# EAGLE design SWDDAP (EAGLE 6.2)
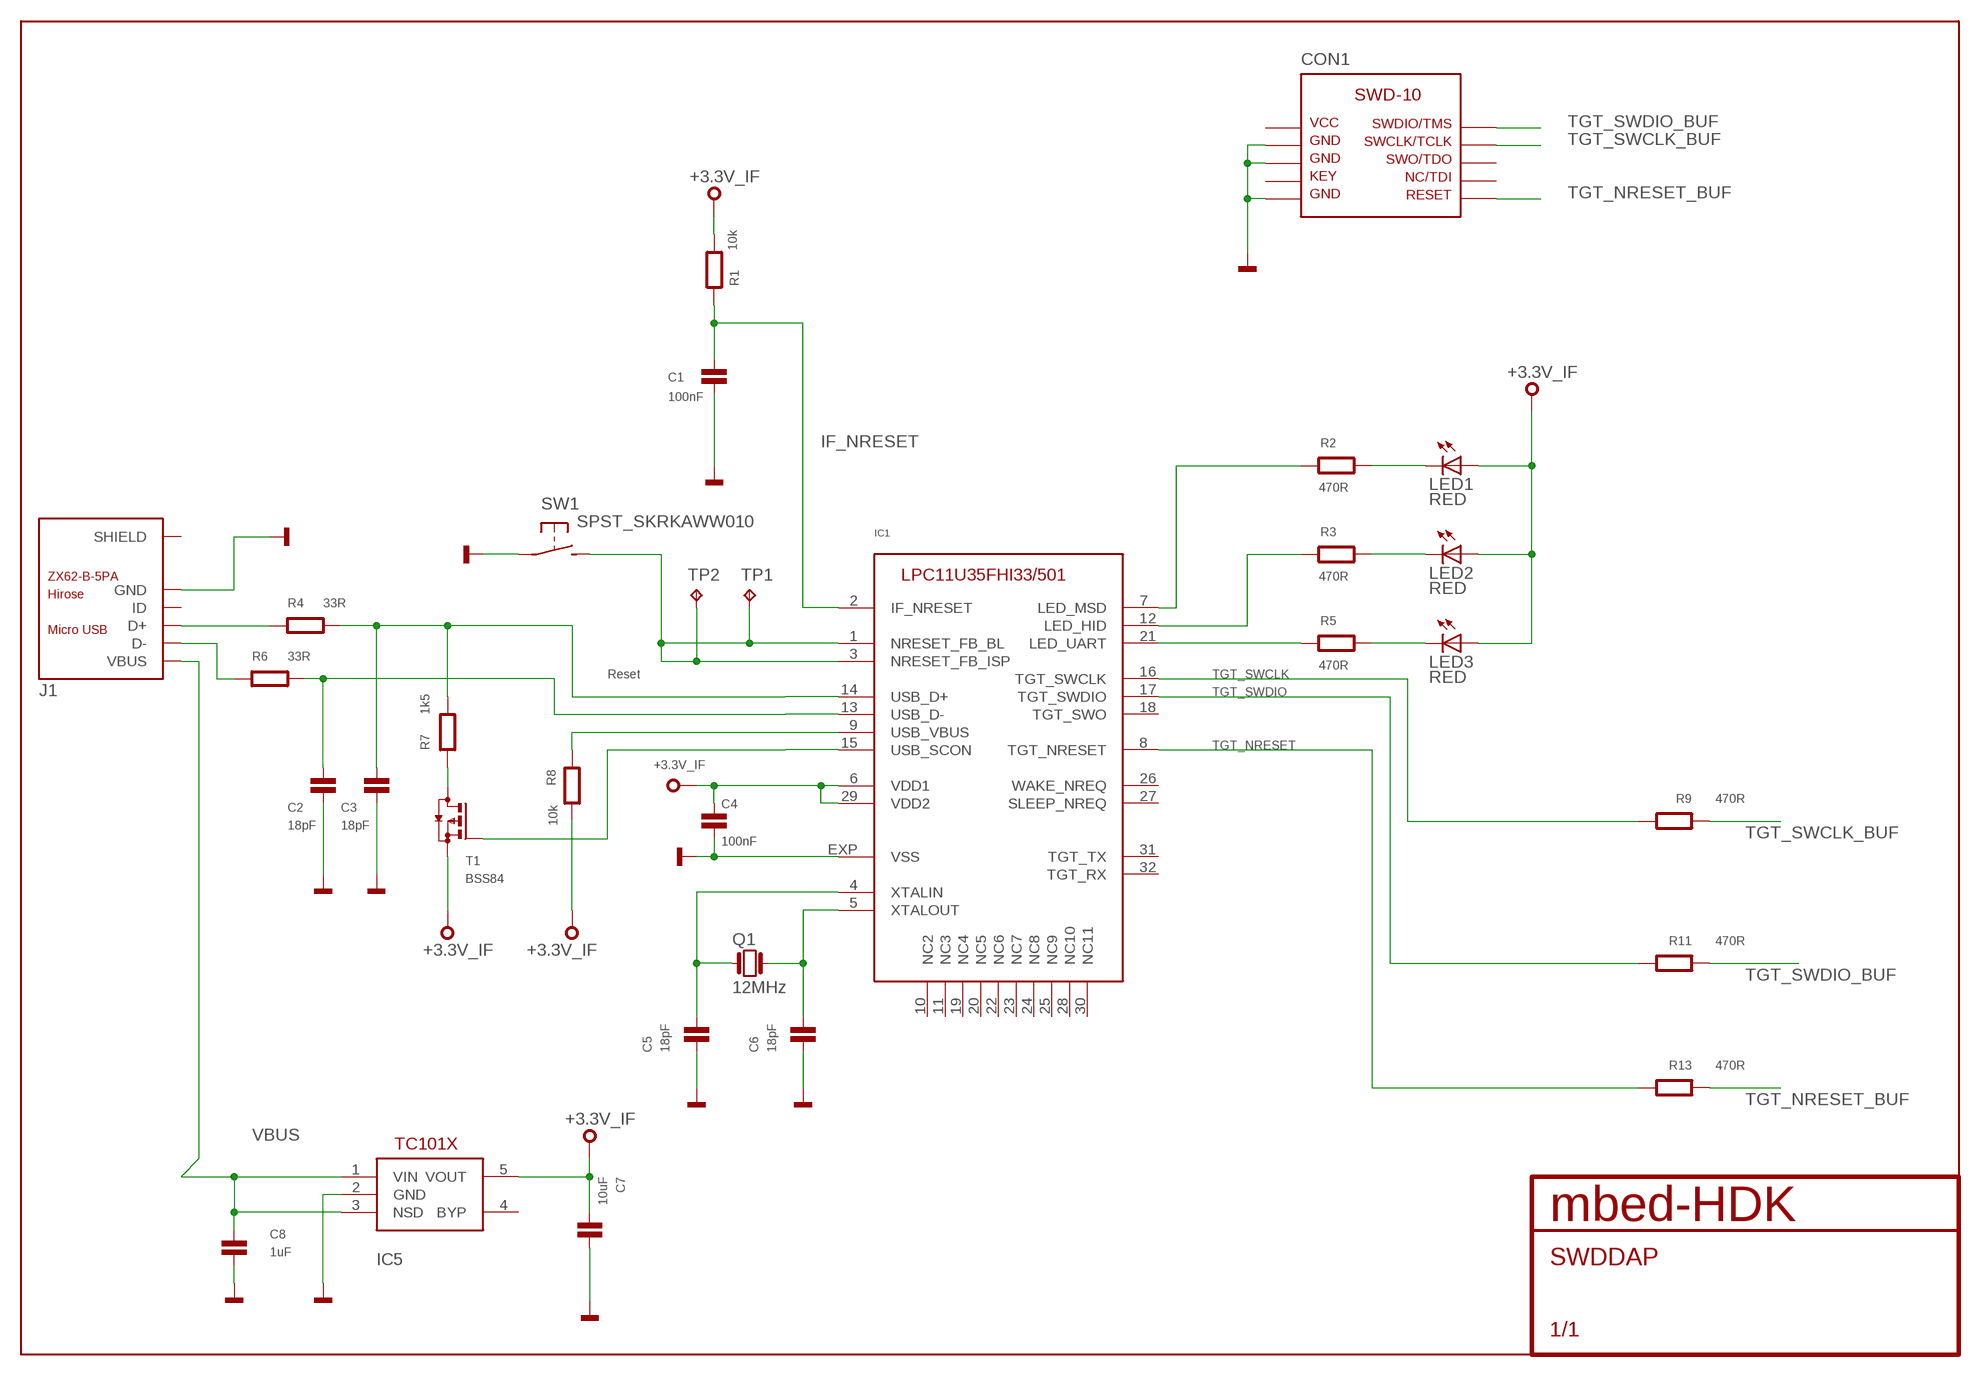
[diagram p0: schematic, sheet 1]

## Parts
C1  100nF  C0402  [0402]
C2  18pF  C0402  [0402]
C3  18pF  C0402  [0402]
C4  100nF  C0402  [0402]
C5  18pF  C0402  [0402]
C6  18pF  C0402  [0402]
C7  10uF  C0603  [0603]
C8  1uF  C0402  [0402]
CON1  SWD-10_SMD  [SWD-10-SMD]
IC1  IF-LPC11U35  [HVQFN33]
IC5  TC1014  [SOT23-5]
J1  ZX62-B-5PA  [ZX62-B-5PA(11)]
LED1  RED  LED0603  [CHIPLED_0603]
LED2  RED  LED0603  [CHIPLED_0603]
LED3  RED  LED0603  [CHIPLED_0603]
Q1  12MHz  Q_3.2X2.5  [3.2X.2.5]
R1  10k  R0402  [0402]
R2  470R  R0402  [0402]
R3  470R  R0402  [0402]
R4  33R  R0402  [0402]
R5  470R  R0402  [0402]
R6  33R  R0402  [0402]
R7  1k5  R0402  [0402]
R8  10k  R0402  [0402]
R9  470R  R0402  [0402]
R11  470R  R0402  [0402]
R13  470R  R0402  [0402]
SW1  SPST_SKRKAWW010  [SKRKAEE010]
T1  BSS84  [SOT23]
TP1  TPTP08SQ  [TP08SQ]
TP2  TPTP08SQ  [TP08SQ]

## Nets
+3,3V: C4.1 C7.2 IC1.6(VDD1) IC1.29(VDD2) IC5.5(VOUT) LED1.A LED2.A LED3.A R1.2 R8.2 T1.2(S) ; supply symbol labelled +3.3V_IF
GND: C1.2 C2.2 C3.2 C4.2 C5.2 C6.2 C7.1 C8.1 CON1.P$3 CON1.P$5 CON1.P$9 IC1.EXP(VSS) IC5.2(GND) J1.5(GND) SW1.P$1(P)
HID: IC1.12(LED_HID) R3.2
IF_NRESET: C1.1 IC1.2(IF_NRESET) R1.1
ISP: IC1.1(NRESET_FB_BL) IC1.3(NRESET_FB_ISP) SW1.P$2(S) TP1.TP TP2.TP
MSD: IC1.7(LED_MSD) R2.2
N$1: C3.1 IC1.14(USB_D+) R4.2 R7.2
N$2: C2.1 IC1.13(USB_D-) R6.2
N$3: J1.2(D-) R6.1
N$4: J1.3(D+) R4.1
N$5: LED1.C R2.1
N$6: R7.1 T1.3(D)
N$7: IC1.9(USB_VBUS) R8.1
N$8: LED2.C R3.1
N$9: LED3.C R5.1
N$12: C6.1 IC1.5(XTALOUT) Q1.P$3
N$14: C5.1 IC1.4(XTALIN) Q1.P$1
N$19: IC1.15(USB_SCON) T1.1(G)
TGT_NRESET: IC1.8(TGT_NRESET) R13.2
TGT_NRESET_BUF: CON1.P$10 R13.1
TGT_SWCLK: IC1.16(TGT_SWCLK) R9.2
TGT_SWCLK_BUF: CON1.P$4 R9.1
TGT_SWDIO: IC1.17(TGT_SWDIO) R11.2
TGT_SWDIO_BUF: CON1.P$2 R11.1
UART: IC1.21(LED_UART) R5.2
VBUS: C8.2 IC5.1(VIN) IC5.3(NSD) J1.1(VBUS)
Unconnected: CON1.P$1 CON1.P$6 CON1.P$7 CON1.P$8 IC1.10(NC2) IC1.11(NC3) IC1.18(TGT_SWO) IC1.19(NC4) IC1.20(NC5) IC1.22(NC6) IC1.23(NC7) IC1.24(NC8) IC1.25(NC9) IC1.26(WAKE_NREQ) IC1.27(SLEEP_NREQ) IC1.28(NC10) IC1.30(NC11) IC1.31(TGT_TX) IC1.32(TGT_RX) IC5.4(BYP) J1.4(ID) J1.SH1(SHIELD) J1.SH2(SHIELD) J1.SH3(SHIELD) J1.SH4(SHIELD) J1.SH5(SHIELD) J1.SH6(SHIELD)

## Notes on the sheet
- Reset

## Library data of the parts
C1-C8 = mbed-HDK:C: Capacitor
CON1 = mbed-HDK:SWD-10
IC1 = mbed-HDK:IF-LPC11U35
IC5 = Karasouli:TC1014
J1 = hirose:ZX62-B-5PA
LED1-LED3 = mbed-HDK:LED: SMD LED
Q1 = mbed-HDK:Q
R1-R9 R11 R13 = mbed-HDK:R
SW1 = mbed-switches:SPST
T1 = mbed-HDK:BSS84: P-CHANNEL MOS FET
TP1 TP2 = testpad:TP: Test pad

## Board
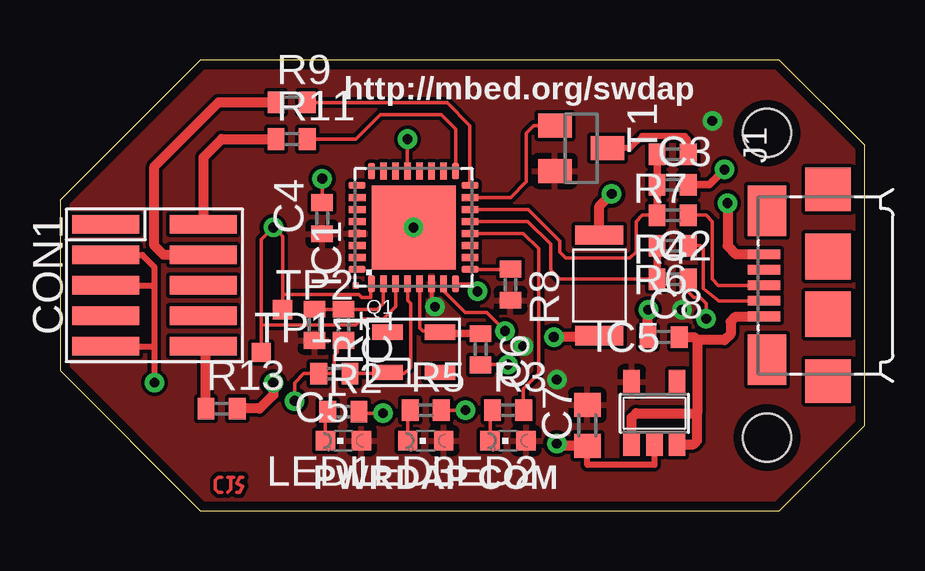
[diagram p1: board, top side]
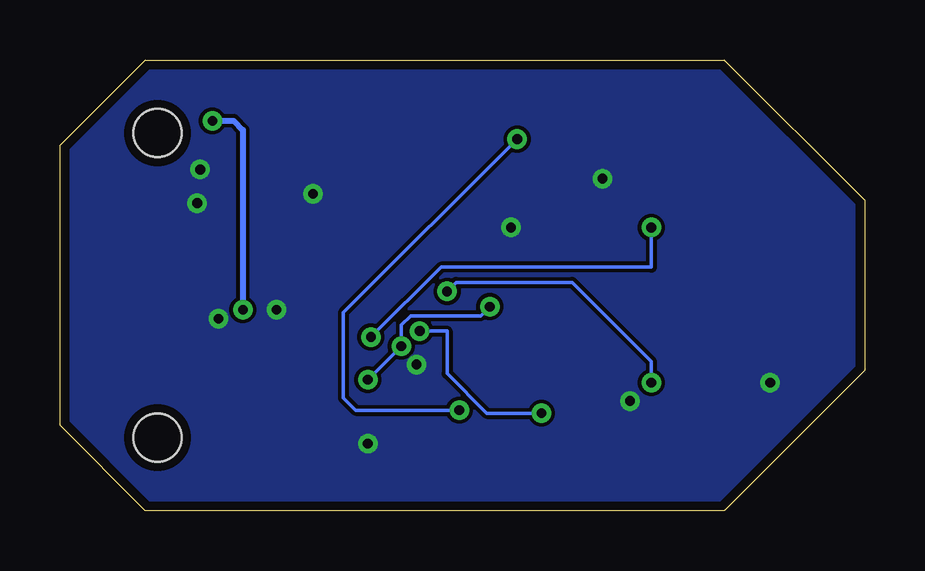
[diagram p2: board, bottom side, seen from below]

Size 33.53 x 18.8 mm. Coordinates in mm from the lower left corner, seen from the top.
Outline: 33.53,3.56 33.53,15.24 29.97,18.8 5.84,18.8 0,12.95 0,5.84 5.84,0 29.97,0 33.53,3.56
Copper layers (1*16): Top 0.035mm / dielectric 1.5mm / Bottom 0.035mm
Design rules: minimum track width 6mil, minimum drill 15mil, track to track 6mil, track to pad 6mil, pad to pad 6mil, via to via 6mil, smd to smd 6mil, copper to edge 15mil, drill to drill 8mil, minimum pad ring 10mil, minimum via ring 8mil, stop-mask expansion 4mil, vias tented up to drill 0mil, thermal gap 10mil
Holes 2 mm at 29.46,3.05 29.46,15.75

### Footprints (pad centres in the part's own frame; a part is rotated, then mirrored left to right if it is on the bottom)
0402 = smd 0.7 x 0.9: 1 -0.65,0; 2 0.65,0
0603 = smd 1 x 1.1: 1 -0.85,0; 2 0.85,0
SWD-10-SMD = smd 0.762 x 2.794: P$1 0.381,-2.032; P$2 0.381,2.032; P$3 1.651,-2.032; P$4 1.651,2.032; P$5 2.921,-2.032; P$6 2.921,2.032; P$7 4.191,-2.032; P$8 4.191,2.032; P$9 5.461,-2.032; P$10 5.461,2.032
HVQFN33 = smd 0.7 x 0.28: 1 -2.35,1.75; 2 -2.35,1.25; 3 -2.35,0.75; 4 -2.35,0.25; 5 -2.35,-0.25; 6 -2.35,-0.75; 7 -2.35,-1.25; 8 -2.35,-1.75; 17 2.35,-1.75; 18 2.35,-1.25; 19 2.35,-0.75; 20 2.35,-0.25; 21 2.35,0.25; 22 2.35,0.75; 23 2.35,1.25; 24 2.35,1.75 | smd 0.28 x 0.7: 9 -1.75,-2.35; 10 -1.25,-2.35; 11 -0.75,-2.35; 12 -0.25,-2.35; 13 0.25,-2.35; 14 0.75,-2.35; 15 1.25,-2.35; 16 1.75,-2.35; 25 1.75,2.35; 26 1.25,2.35; 27 0.75,2.35; 28 0.25,2.35; 29 -0.25,2.35; 30 -0.75,2.35; 31 -1.25,2.35; 32 -1.75,2.35 | smd 3.5 x 3.5: EXP 0,0 | smd 0.25 x 0.25: M1 -2.415,2.415
SOT23-5 = smd 0.69 x 0.99: 1 -0.95,-1.29; 2 0,-1.29; 3 0.95,-1.29; 4 0.95,1.3; 5 -0.95,1.3
ZX62-B-5PA(11) = smd 0.4 x 1.35: 1 -1.3,2.675; 2 -0.65,2.675; 3 0,2.675; 4 0.65,2.675; 5 1.3,2.675 | smd 2.1 x 1.6: SH1 -3.1,2.55; SH2 3.1,2.55 | smd 1.8 x 1.9: SH3 -4,0; SH6 4,0 | smd 1.9 x 1.9: SH4 -1.2,0; SH5 1.2,0
CHIPLED_0603 = smd 0.8 x 0.8: A 0,-0.75; C 0,0.75
3.2X.2.5 = smd 1.27 x 0.635: P$1 -1.092,-0.838; P$2 1.092,-0.838; P$3 1.092,0.838; P$4 -1.092,0.838
SKRKAEE010 = smd 0.8 x 2: P$1 -2.1,0; P$2 2.1,0
SOT23 = smd 1 x 1.4: 1 -0.95,-1.1; 2 0.95,-1.1; 3 0,1.1
TP08SQ = smd 0.8 x 0.8: TP 0,0

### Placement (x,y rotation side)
C1  11.81,7.75 270 top
C2  25.53,9.65 0 top
C3  25.53,13.59 0 top
C4  10.92,12.19 90 top
C5  11.43,5.71 180 top
C6  17.53,6.73 270 top
C7  21.97,3.56 90 top
C8  25.15,7.24 0 top
CON1  3.94,12.32 270 top
IC1  14.73,11.81 90 top
IC5  24.77,4.06 0 top
J1  32,9.4 90 top
LED1  11.81,2.92 90 top
LED2  18.67,2.92 90 top
LED3  15.24,2.92 90 top
Q1  14.73,6.6 0 top
R1  10.6,7.75 270 top
R2  11.81,4.13 0 top
R3  18.67,4.19 0 top
R4  25.53,12.32 180 top
R5  15.24,4.19 0 top
R6  25.53,11.05 180 top
R7  25.53,14.86 180 top
R8  18.77,9.42 270 top
R9  9.65,17.02 0 top
R11  9.65,15.49 0 top
R13  6.73,4.25 0 top
SW1  22.48,9.4 270 top
T1  21.72,15.11 270 top
TP1  8.38,6.6 0 top
TP2  9.27,8.38 0 top

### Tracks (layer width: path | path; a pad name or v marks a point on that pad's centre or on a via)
+3,3V  (via drill 0.41)
  Top 0.152: IC1.6 15.48,8.65 v15.62,8.51
  Bottom 0.152: v15.62,8.51 16,8.13 18.92,8.13 19.3,7.75 v19.3,6.86 v20.7,5.46
  Bottom 0.254: v27.18,16.26 26.29,16.26 25.91,15.88 v25.91,8.38
  pour Top: -5.08,19.18 -5.08,-0.25 34.54,-0.25 34.54,19.18
GND  (via drill 0.41)
  Top 0.152: C1.2 11.56,6.84 11.56,6.6 11.43,6.48 11.43,5.84 11.3,5.71 C5.2 10.16,5.71 9.78,5.33 v9.78,4.57 | C4.2 v10.92,13.84 10.68,14.08 | C6.2 17.54,6.1 v18.67,6.1 | C2.2 26.18,9.13 26.42,8.89 26.67,8.89 26.92,8.64 v26.92,8
  Top 0.254: IC5.2 24.77,1.9 21.97,1.9 C7.1 | CON1.P$3 3.43,10.67 3.94,10.16 3.94,9.4 | 3.94,9.4 3.94,6.86 | 3.94,6.86 v3.94,5.33 | CON1.P$9 3.94,6.86 | CON1.P$5 3.94,9.4
  Top 0.305: v27.69,14.22 27.05,13.59 C3.2
  Top 0.406: C7.1 20.7,2.71 v20.7,2.79 | C7.1 22.1,2.71 | 22.01,2.67 C7.1 | C8.1 24.5,8.37 v24.51,8.38 | 27.81,14.1 v27.69,14.22 | v27.81,12.83 27.81,11.05 28.16,10.7 J1.5 | SW1.P$1 22.48,12.7 v22.99,13.21
  other vias: 14.73,11.81
  pour Bottom: -5.08,-0.25 34.54,-0.25 34.54,19.18 -5.08,19.18
HID
  Top 0.152: IC1.12 19.3,11.56 19.94,10.92 19.94,5.71 19.3,5.08 19.3,4.21 R3.2
IF_NRESET
  Top 0.152: R1.1 C1.1 13.22,8.4 13.46,8.64 13.46,9.44 IC1.2
ISP  (via drill 0.41)
  Top 0.152: IC1.1 12.95,9.46 12.95,8.89 12.57,8.89 12.45,9.02 9.27,9.02 | IC1.3 13.98,8.52 13.46,8 12.57,8 12.32,7.75 8.38,7.75 | 8.38,7.75 8.38,11.3 v8.89,11.81 9.27,11.43 9.27,9.02 | TP1.TP 8.38,7.75 | TP2.TP 9.27,9.02
  Top 0.406: SW1.P$2 22.42,7.24 v20.57,7.24
  Bottom 0.152: v8.89,11.81 8.89,10.16 17.65,10.16 v20.57,7.24
MSD  (via drill 0.41)
  Top 0.152: IC1.7 15.98,9.16 16.89,8.25 17.78,8.25 v18.54,7.49 | v13.46,4.06 12.53,4.06 R2.2
  Bottom 0.152: v18.54,7.49 17.4,7.49 17.4,5.71 15.75,4.06 v13.46,4.06
N$1
  Top 0.152: IC1.14 19.51,12.56 20.83,11.24 20.83,10.79 21.08,10.54 23.75,10.54 24,10.79 24,12.06 24.26,12.32 R4.2
  Top 0.305: R4.2 C3.1 R7.2
N$2
  Top 0.152: IC1.13 19.5,12.06 20.45,11.11 20.45,10.03 20.83,9.65 C2.1
  Top 0.305: R6.2 C2.1
N$3
  Top 0.152: R6.1 26.67,11.05 26.8,10.92 26.8,9.91 26.8,9.78 26.8,9.27 27.43,8.76 27.45,8.75 J1.2
N$4
  Top 0.152: R4.1 26.92,12.32 27.18,12.06 27.18,9.65 27.43,9.4 J1.3
N$5
  Top 0.152: LED1.C 11.06,3.9 R2.1
N$6
  Top 0.254: R7.1 26.18,15.48 26.03,15.62 24.26,15.62 23.75,15.11 T1.3
N$7
  Top 0.152: IC1.9 18.76,10.06 R8.1
N$8
  Top 0.152: LED2.C 17.92,4.09 R3.1
N$9
  Top 0.152: LED3.C 14.49,4.09 R5.1
N$11
  Top 0.152: 6.73,1.4 6.6,1.4 6.48,1.27 6.48,0.89 6.6,0.76 6.73,0.76
N$12
  Top 0.152: IC1.5 14.98,7.62 15.11,7.49 15.77,7.49 Q1.P$3
  Top 0.305: Q1.P$3 15.88,7.38 C6.1
N$13
  Top 0.152: 6.99,1.4 7.11,1.4 | 7.11,1.4 7.24,1.4 | 7.11,1.4 7.11,0.89 6.99,0.76
N$14
  Top 0.152: IC1.4 14.48,8.76 14.6,8.64 14.61,5.97 14.35,5.71 13.69,5.71 Q1.P$1 13.59,5.71 C5.1
N$15
  Top 0.152: 7.62,1.4 7.49,1.4 7.37,1.14 7.62,1.02 7.49,0.76 7.37,0.76
N$19
  Top 0.152: IC1.15 18.78,13.06 19.43,13.72 19.43,15.75 19.69,16 19.75,16.06 T1.1
TGT_NRESET  (via drill 0.41)
  Top 0.152: IC1.8 17.08,9.46 v17.4,9.14
  Top 0.406: v8.89,5.33 8.89,4.83 8.32,4.25 R13.2
  Bottom 0.152: v17.4,9.14 17.02,9.53 12.19,9.53 8.89,6.22 v8.89,5.33
TGT_NRESET_BUF
  Top 0.406: 6.03,6.79 CON1.P$10 6.08,6.75 R13.1
TGT_SWCLK
  Top 0.152: IC1.16 17.08,16.06 16.13,17.02 R9.2
TGT_SWCLK_BUF
  Top 0.406: CON1.P$4 4.32,10.67 3.94,11.05 3.94,14.35 6.6,17.02 R9.1
TGT_SWDIO
  Top 0.152: IC1.17 16.48,15.9 15.87,16.51 13.33,16.51 12.32,15.49 R11.2
TGT_SWDIO_BUF
  Top 0.406: CON1.P$2 5.97,14.73 6.73,15.49 R11.1
UART  (via drill 0.41)
  Top 0.152: IC1.21 v14.48,15.49 | v16.89,4.19 R5.2
  Bottom 0.152: v14.48,15.49 21.72,8.25 21.72,4.7 21.21,4.19 v16.89,4.19
VBUS
  Top 0.406: IC5.1 23.81,3.88 24,4.06 26.54,4.06 | IC5.3 26.4,2.77 26.54,2.92 26.54,3.81 26.54,4.06 | C8.2 26.42,7.24 26.54,7.11 | 26.54,7.11 26.54,4.06 | 26.54,7.11 27.69,7.11 27.94,7.37 27.94,7.87 28.16,8.1 J1.1

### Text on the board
TopSilkscreen: http://mbed.org/swdap | PWR | DAP | COM
BottomSilkscreen: http://mbed.org/swdap | USB CMSIS-DAP Interface | for Serial Wire Debug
